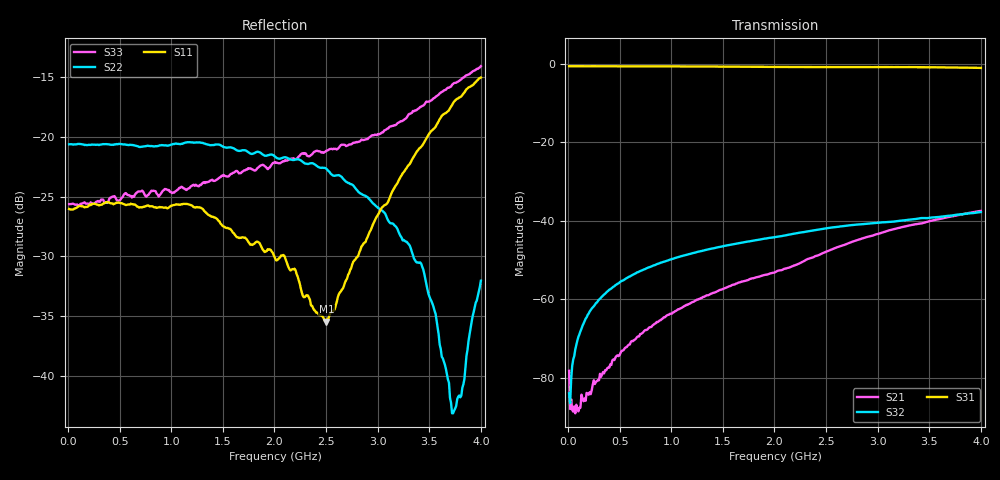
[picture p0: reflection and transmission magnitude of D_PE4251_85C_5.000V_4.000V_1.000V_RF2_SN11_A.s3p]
! Device ID: PE4251_SoldCshunt_081809
! Dir: c:\Test Bench Repositories\Bench_Software_CVI_Version_8\trunk\PSC 4Port_VNA Bench\datalog\4250\TEST\PE4251_SoldCshunt_081809\85C\5p000000\RF2
! Serial: 11
! Insertion: A
! Temp: 85C
! VDD: 5.000
! Control_Hi: 80.000
! Control_Lo: 20.000
! Logic State: RF2
! Port 1: RFC
! Port 2: RF1
! Port 3: RF2
! V1 = 1.00
! V2 = 1.00
! V3 = 1.00
! IDD: 6.371300e-05
! FILE NAME
! DATE 08/18/09  20:18
! CORRECTED  DATA
#  Hz  S  RI  R  50.00
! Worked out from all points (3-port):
!   401 points, 10 MHz to 4 GHz, reference 50 ohm
!   strongest paths, dB at 10 MHz, 1.008 GHz, 2.005 GHz, 3.002 GHz, 4 GHz:
!     S31: -0.6, -0.7, -0.8, -0.8, -1.0
!     S32: -83.9, -49.7, -44.1, -40.5, -37.7
!     S21: -78.2, -63.6, -53.1, -43.3, -37.4
!   lowest |S11| = -35.5 dB at 2.504 GHz (marker M1), VSWR 1.03, Z = 50.4 - j1.64 ohm
!   |S11| at or under -10 dB: start of sweep to end of sweep
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1e7  0.0499 -0.000464  1.66e-05 5.55e-05  0.9312 -0.00369
     0.000124 4.99e-06  0.0932 -0.000898  8.75e-05 5.74e-05
     0.9319 -0.00439  -5.34e-05 3.51e-05  0.0523 0.000506
1.79575e8  0.0509 0.000245  5.06e-06 -4.83e-05  0.9291 -0.0638
           5.38e-06 -6.44e-05  0.0924 -0.0042  5.42e-05 0.000589
           0.929 -0.0635  5.96e-05 0.000589  0.0525 -0.000721
3.0925e8  0.0519 -0.00153  -3.69e-05 -8.64e-05  0.9237 -0.1087
          -4.07e-05 -0.000106  0.0925 -0.00803  8.88e-05 0.00103
          0.9248 -0.1082  9.41e-05 0.00101  0.0535 -0.00291
4.98775e8  0.0528 -0.00378  -0.00015 -0.000139  0.9125 -0.1722
           -0.00014 -0.000136  0.0928 -0.0121  0.000158 0.00163
           0.9124 -0.172  0.000156 0.00164  0.054 -0.00487
1.1272e9  0.0509 -0.0127  -0.000798 -0.000146  0.8471 -0.3725
          -0.000813 -0.000147  0.09 -0.0283  0.000524 0.00361
          0.8481 -0.3725  0.000518 0.0036  0.0591 -0.0145
2.005e9  0.0302 -0.00727  -0.00223 -8.19e-05  0.6863 -0.6027
         -0.00222 -7.79e-05  0.0764 -0.0318  0.00105 0.00614
         0.6876 -0.6036  0.00105 0.00616  0.0686 -0.0382
2.50375e9  0.00429 -0.0162  -0.00405 -0.000378  0.5749 -0.7007
           -0.00406 -0.000381  0.0675 -0.029  0.00138 0.00793
           0.5769 -0.7008  0.0014 0.00795  0.0502 -0.0719
3.42145e9  -0.0823 -0.0389  -0.00909 0.00194  0.3241 -0.8453
           -0.0091 0.00192  0.0239 -0.0172  0.00202 0.0106
           0.3265 -0.8449  0.00203 0.0107  -0.0356 -0.1292
3.730675e9  -0.1335 -0.0377  -0.011 0.00341  0.2163 -0.8691
            -0.011 0.0034  -0.000477 -0.00693  0.00189 0.0116
            0.2173 -0.8696  0.00188 0.0116  -0.0896 -0.1407
4e9  -0.175 -0.0301  -0.0125 0.00506  0.1177 -0.8793
     -0.0125 0.00503  -0.0249 -0.00181  0.00195 0.0128
     0.119 -0.8783  0.00196 0.0128  -0.1419 -0.1381
